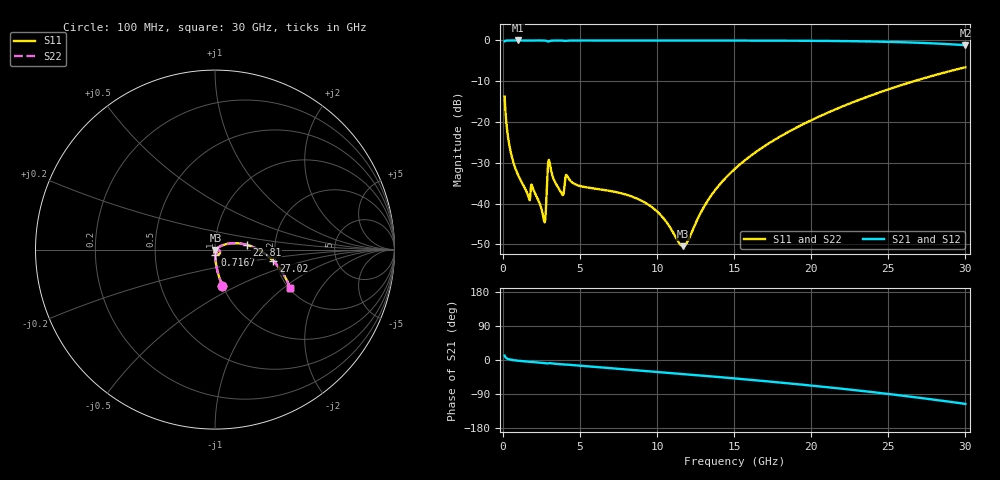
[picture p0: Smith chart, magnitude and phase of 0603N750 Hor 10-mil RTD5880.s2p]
# GHz S MA R 50
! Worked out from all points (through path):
!   3201 points, 100 MHz to 30 GHz, reference 50 ohm
!   highest |S21| = -0.01 dB at 987.7 MHz (marker M1); lowest = -1.2 dB at 30 GHz (marker M2)
!   group delay of S21, straight-line fit = 10.5 ps
!   lowest |S11| = -50.4 dB at 11.68 GHz (marker M3), VSWR 1.01, Z = 50.2 - j0.19 ohm
!   |S11| at or under -10 dB: start of sweep to 26.66 GHz
!   |S22| runs from -50.4 to -6.6 dB; largest |S21 - S12| = 0
!   S11 on the Smith chart (normalised r, x): 100 MHz: 1.00, -0.42; 716.7 MHz: 1.00, -0.06; 22.81 GHz: 1.42, +0.08; 27.02 GHz: 1.94, -0.28; 30 GHz: 2.03, -1.10
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0.1  0.2053 -78.4  0.9783 11.5  0.9783 11.5  0.2053 -78.4
0.3896562  0.05415 -87.6  0.998 1.8  0.998 1.8  0.05415 -87.6
0.7166875  0.02998 -89.3  0.9989 -0.6  0.9989 -0.6  0.02998 -89.3
0.9876563  0.02213 -89.9  0.9989 -1.9  0.9989 -1.9  0.02213 -89.9
1.623031  0.01247 -86.5  0.9982 -4.5  0.9982 -4.5  0.01247 -86.5
1.959406  0.01497 -85.9  0.9974 -5.5  0.9974 -5.5  0.01497 -85.9
2.632156  0.006488 -65.9  0.9965 -8.2  0.9965 -8.2  0.006488 -65.9
2.725594  0.006157 -31.6  0.9943 -8.7  0.9943 -8.7  0.006157 -31.6
3.024594  0.03138 -65.8  0.9828 -8.2  0.9828 -8.2  0.03138 -65.8
3.790781  0.01333 -84.6  0.996 -11.5  0.996 -11.5  0.01333 -84.6
4.164531  0.02177 -84.9  0.9932 -12.2  0.9932 -12.2  0.02177 -84.9
5.089563  0.01625 -97.9  0.9977 -15.4  0.9977 -15.4  0.01625 -97.9
8.238406  0.01242 -104.4  0.9974 -25.6  0.9974 -25.6  0.01242 -104.4
10.06978  0.007752 -101.1  0.9971 -31.6  0.9971 -31.6  0.007752 -101.1
11.67691  0.003004 -39.0  0.9968 -37.0  0.9968 -37.0  0.003004 -39.0
13.41484  0.01187 30.7  0.9964 -42.9  0.9964 -42.9  0.01187 30.7
15.05  0.02673 33.4  0.9958 -48.7  0.9958 -48.7  0.02673 33.4
20.03956  0.106 19.6  0.9891 -67.6  0.9891 -67.6  0.106 19.6
22.81466  0.1779 8.6  0.9778 -79.5  0.9778 -79.5  0.1779 8.6
25.01978  0.2517 -1.3  0.9606 -89.7  0.9606 -89.7  0.2517 -1.3
27.01934  0.3314 -11.1  0.9354 -99.7  0.9354 -99.7  0.3314 -11.1
30  0.4683 -27.0  0.874 -115.9  0.874 -115.9  0.4683 -27.0
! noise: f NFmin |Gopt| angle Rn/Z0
0.1  0.000283  0.9159  0.3694  0.0007421
3.417  0.004836  0.839  11.03  0.006303
6.743  0.005703  0.7464  21.67  0.004366
10.06  0.007691  0.7264  32.04  0.005173
13.39  0.009755  0.7192  42.15  0.006011
16.7  0.01195  0.7197  51.87  0.006871
20.03  0.01439  0.7261  61.21  0.0078
23.35  0.01716  0.737  70.13  0.00884
26.67  0.02042  0.7518  78.68  0.01006
30  0.02438  0.7697  86.86  0.01154
